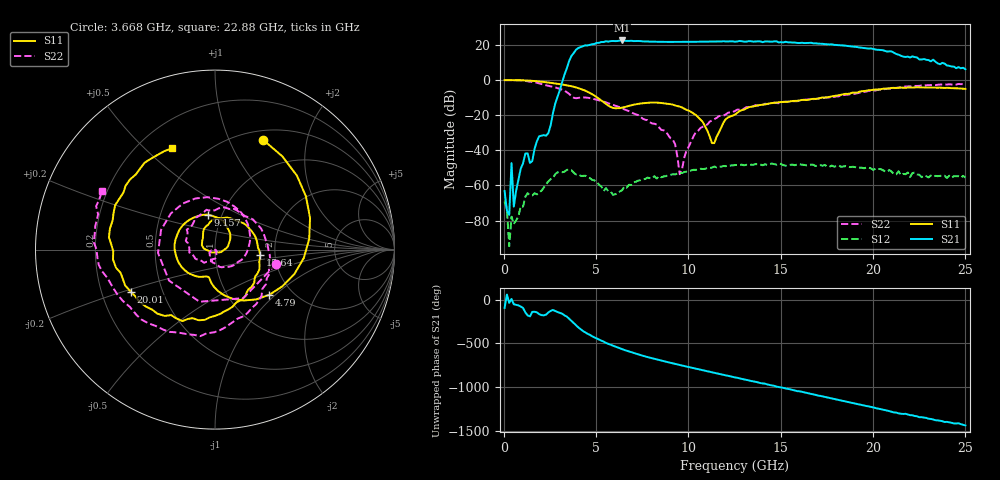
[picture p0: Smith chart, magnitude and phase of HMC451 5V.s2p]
!Hittite Microwave Corporation
!20 Alpha Road
!Chelmsford, MA 01824
!Tel: 978-250-3343
!Fax: 978-250-3373
!Device: HMC451, 5-20 GHz, Driver Amplifier Die
!Misc: Vcc = 5V, room. Die measured in housing that includes two K connectors, not de-embedded.
# MHZ S MA R 50
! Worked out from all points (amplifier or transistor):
!   201 points, 50 MHz to 25 GHz, reference 50 ohm
!   highest |S21| = 22.5 dB at 6.412 GHz (marker M1)
!   |S21| within 3 dB of that: 4.362 GHz to 18.49 GHz (14.12 GHz wide, 124 % of centre)
!   unconditionally stable (mu >= 1): start of sweep to end of sweep
!   at 4.167 GHz: K = 19.36, MAG = 20.8 dB, |S12| = -54.6 dB
!   at 12.53 GHz: K = 10.39, MAG = 21.9 dB, |S12| = -48.4 dB
!   at 25 GHz: K = 43.28, MAG = 11.5 dB, |S12| = -55.6 dB
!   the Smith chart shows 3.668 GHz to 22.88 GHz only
!   S11 on the Smith chart (normalised r, x): 3.668 GHz: 0.61, +1.35; 4.79 GHz: 1.54, -0.92; 9.157 GHz: 0.86, +0.35; 15.64 GHz: 1.67, -0.11; 20.01 GHz: 0.33, -0.21; 22.88 GHz: 0.34, +0.61
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50  0.995 -3.5  0.0006912 -95.2  0.0003477 -32.5  0.995 -3.8
3168.75  0.745 112.1  0.884 -161.4  0.002371 96.0  0.529 97.8
3667.75  0.667 66.2  4.826 115.6  0.002728 56.2  0.35 -13.3
3917.25  0.615 42.1  7.27 66.9  0.002044 31.9  0.303 -106.5
4291.5  0.528 6.4  9.182 0.9  0.001857 19.5  0.32 159.9
4790.5  0.394 -39.7  10.41 -59.9  0.001442 6.4  0.295 98.3
5414.25  0.232 -85.6  12.09 -121.2  0.0006932 -6.0  0.243 46.4
5913.25  0.161 -101.4  12.93 -167.1  0.000542 22.8  0.197 11.1
6412.25  0.163 -112.3  13.36 153.2  0.0007305 45.4  0.159 -20.8
7285.5  0.21 -152.9  12.92 93.4  0.001368 45.6  0.1 -74.6
8408.25  0.225 144.1  12.22 29.0  0.001839 26.7  0.045 -128.9
9156.75  0.199 102.0  12.12 -9.3  0.002068 24.7  0.02 -170.7
10778.5  0.064 7.0  12.36 -87.7  0.002922 1.4  0.047 -86.1
12525  0.104 130.0  12.34 -170.0  0.003803 -30.5  0.131 -169.9
14271.5  0.208 47.5  12.52 109.8  0.003836 -66.6  0.207 118.7
15643.75  0.253 -6.7  11.64 46.5  0.003906 -87.2  0.25 60.7
16766.5  0.291 -45.5  11.03 -4.7  0.003883 -111.2  0.286 15.7
18388.25  0.395 -98.1  9.636 -79.2  0.003454 -141.6  0.371 -48.0
20010  0.525 -153.5  7.677 -153.3  0.002761 -176.0  0.497 -108.8
20883.25  0.578 177.3  6.548 164.5  0.002742 166.6  0.569 -140.4
22879.25  0.613 113.0  3.781 87.4  0.001834 140.3  0.708 152.6
25000  0.559 49.5  2.022 0.7  0.001668 113.9  0.756 86.9
